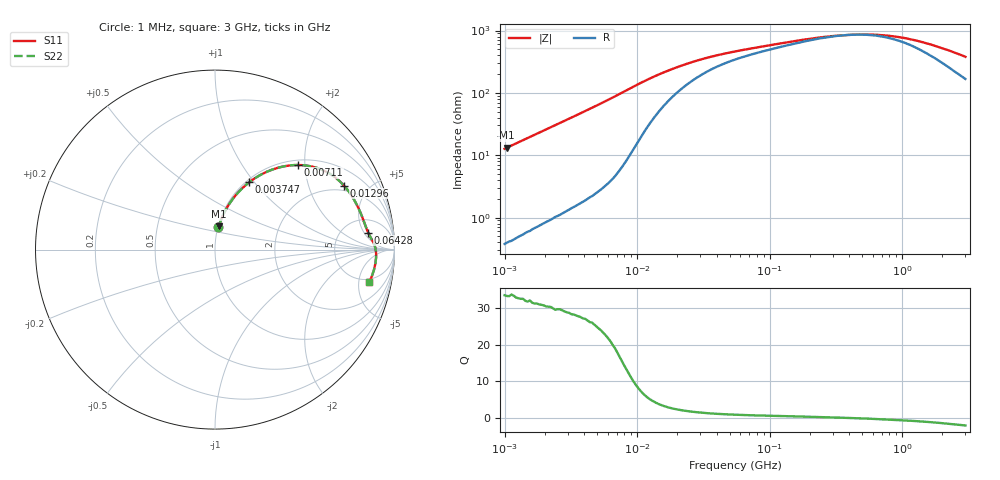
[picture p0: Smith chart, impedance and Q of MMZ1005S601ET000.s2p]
! S-parameter Generated by TDK Corporation
! Copyright(C) 2016 TDK Corporation.
! All Rights Reserved.
! TDK P/N: MMZ1005S601ET000 (Chip Beads)
! Property: |Z|=600¶ at 100MHz
! Size(LxWxT): 1x0.5x0.5mm, 0.039x0.02x0.02inches
! Model Type: s2p (Touchstone File Format Version 1.0)
! Frequency: DC=Yes Start=1MHz Stop=3000MHz 202points Log-sweep
! Note: This model was converted from impedance.
! Model Generated on May. 16, 2016
! Hash(MD5):
! Port Assignments:
!  1 ---@@@--- 2
! Applicable Conditions:
!  Temperature = 25 degC
!  DC Bias Current = 0 A
!  Small Signal Operation
! Terms and conditions regarding TDK Simulation Models
! (1)This simulation model is being provided solely for informational purposes. Please refer to the specifications of the products in terms of detailed characteristics of such products.
! (2)In no event shall TDK Corporation of any of its subsidiaries be liable for any loss or damage arising, directly or indirectly,
!  From any information contained in this simulation model, including, but not limited to loss or damages arising from any inaccuracies, omissions or errors in connection with such information.
! (3)Any and all copyrights on this simulation model are owned by TDK Corporation.
!  Duplication or redistribution of this simulation model without prior written permission from TDK Corporation is prohibited.
! (4)This simulation model is subject to any modification or change without any prior notice.
! (5)Neither TDK Corporation nor any of its subsidiaries shall make any warranty, express or implied,
!  Including but not limited to the correctness, implied warranties of merchantability and fitness for a particular purpose with respect to this simulation models.
! (6)The use of this simulation model shall be deemed to have consented to the terms and conditions hereof.
# MHz S MA R 50
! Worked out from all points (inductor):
!   201 points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, 1 MHz to 3 GHz, reference 50 ohm
!   read as one part in series: L = 2.02 uH near 1.041 MHz
!   highest Q = 33.6 at 1.041 MHz (marker M1), where L = 2.02 uH
!   self-resonance near 412.7 MHz
!   S11 on the Smith chart (normalised r, x): 1 MHz: 1.01, +0.25; 3.747 MHz: 1.03, +0.94; 7.11 MHz: 1.10, +1.84; 12.96 MHz: 1.73, +3.46; 64.28 MHz: 9, +6; 3 GHz: 4.35, -6.79
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1  0.1255 81.1  0.9884 -7.2  0.9884 -7.2  0.1255 81.1
1.040844  0.1306 80.8  0.9875 -7.5  0.9875 -7.5  0.1306 80.8
2.13957  0.2584 73.2  0.9576 -15.0  0.9576 -15.0  0.2584 73.2
2.83156  0.332 68.7  0.932 -19.4  0.932 -19.4  0.332 68.7
3.747356  0.4207 63.1  0.8921 -24.9  0.8921 -24.9  0.4207 63.1
3.900413  0.4345 62.2  0.8849 -25.7  0.8849 -25.7  0.4345 62.2
5.372736  0.553 54.1  0.8104 -33.5  0.8104 -33.5  0.553 54.1
7.110411  0.6599 45.6  0.7152 -41.2  0.7152 -41.2  0.6599 45.6
9.040831  0.7378 37.5  0.6113 -47.3  0.6113 -47.3  0.7378 37.5
10.61086  0.7744 32.2  0.5379 -50.1  0.5379 -50.1  0.7744 32.2
12.9622  0.8024 26.4  0.4542 -51.7  0.4542 -51.7  0.8024 26.4
14.61624  0.8129 23.4  0.4107 -51.8  0.4107 -51.8  0.8129 23.4
19.34349  0.8281 17.8  0.3295 -50.1  0.3295 -50.1  0.8281 17.8
27.73354  0.8397 12.7  0.2581 -45.5  0.2581 -45.5  0.8397 12.7
54.77226  0.855 7.1  0.1852 -35.0  0.1852 -35.0  0.855 7.1
64.28402  0.8586 6.3  0.1745 -32.8  0.1745 -32.8  0.8586 6.3
213.6344  0.8866 2.1  0.1183 -15.6  0.1183 -15.6  0.8866 2.1
439.1493  0.8958 -0.2  0.1042 1.7  0.1042 1.7  0.8958 -0.2
800.5644  0.8984 -2.4  0.1093 20.4  0.1093 20.4  0.8984 -2.4
1147.801  0.8978 -4.2  0.1233 32.0  0.1233 32.0  0.8978 -4.2
1519.029  0.8956 -5.9  0.1429 40.2  0.1429 40.2  0.8956 -5.9
3000  0.8759 -12.0  0.2314 51.8  0.2314 51.8  0.8759 -12.0
